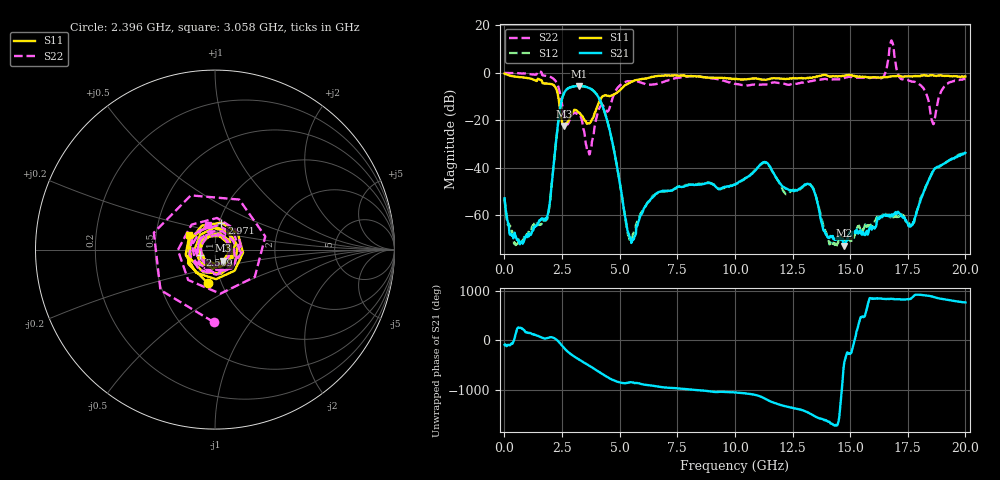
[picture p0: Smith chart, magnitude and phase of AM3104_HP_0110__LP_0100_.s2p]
!Created with skrf (http://scikit-rf.org).
# Hz S RI R 50.0
!freq ReS11 ImS11 ReS21 ImS21 ReS12 ImS12 ReS22 ImS22
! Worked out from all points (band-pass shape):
!   1601 points, 10 MHz to 20 GHz, reference 50 ohm
!   highest |S21| = -5.50 dB at 3.246 GHz (marker M1); lowest = -72.7 dB at 14.75 GHz (marker M2)
!   |S21| within 3 dB of the highest: 2.589 GHz to 3.958 GHz (1.369 GHz wide, 41.8 % of centre)
!   lowest |S11| = -22.3 dB at 2.584 GHz (marker M3), VSWR 1.17, Z = 54.5 - j6.66 ohm
!   |S11| at or under -10 dB: 2.337 GHz to 4.245 GHz (1.908 GHz wide, 58 % of centre)
!   |S22| runs from -34.3 to 13.6 dB; largest |S21 - S12| = 0.029
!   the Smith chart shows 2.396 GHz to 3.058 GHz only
!   S11 on the Smith chart (normalised r, x): 2.396 GHz: 0.86, -0.34; 2.509 GHz: 0.85, -0.05; 2.971 GHz: 1.02, +0.31; 3.058 GHz: 0.74, +0.13
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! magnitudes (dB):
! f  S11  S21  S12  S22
! 10 MHz  -0.3  -52.8  -53.1  0.0
! 509.8 MHz  -1.6  -69.5  -72.2  -0.1
! 1.809 GHz  -4.5  -61.9  -62.1  -1.2
! 2.396 GHz  -14.3  -16.3  -16.3  -7.9
! 2.509 GHz  -21.1  -10.6  -10.7  -13.7
! 2.584 GHz  -22.3  -8.6  -8.6  -17.9
! 2.971 GHz  -16.2  -5.7  -5.8  -17.2
! 3.058 GHz  -15.7  -5.7  -5.7  -16.8
! 3.246 GHz  -16.9  -5.5  -5.6  -17.8
! 3.346 GHz  -17.9  -5.6  -5.7  -19.3
! 3.683 GHz  -21.3  -6.4  -6.5  -34.3
! 4.37 GHz  -9.4  -17.1  -17.2  -15.3
! 5.445 GHz  -4.1  -69.2  -70.0  -3.5
! 6.682 GHz  -1.2  -50.3  -50.2  -4.5
! 10.01 GHz  -2.7  -47.1  -47.1  -4.6
! 13.34 GHz  -2.1  -47.9  -47.7  -3.5
! 14.09 GHz  -1.5  -69.4  -71.7  -2.9
! 14.75 GHz  -1.2  -72.7  -70.9  -2.2
! 16.68 GHz  -1.6  -60.3  -60.1  7.2
! 17.66 GHz  -1.5  -64.2  -64.4  -3.7
! 18.59 GHz  -1.0  -41.6  -41.7  -21.2
! 20 GHz  -1.5  -33.7  -33.4  -2.5
